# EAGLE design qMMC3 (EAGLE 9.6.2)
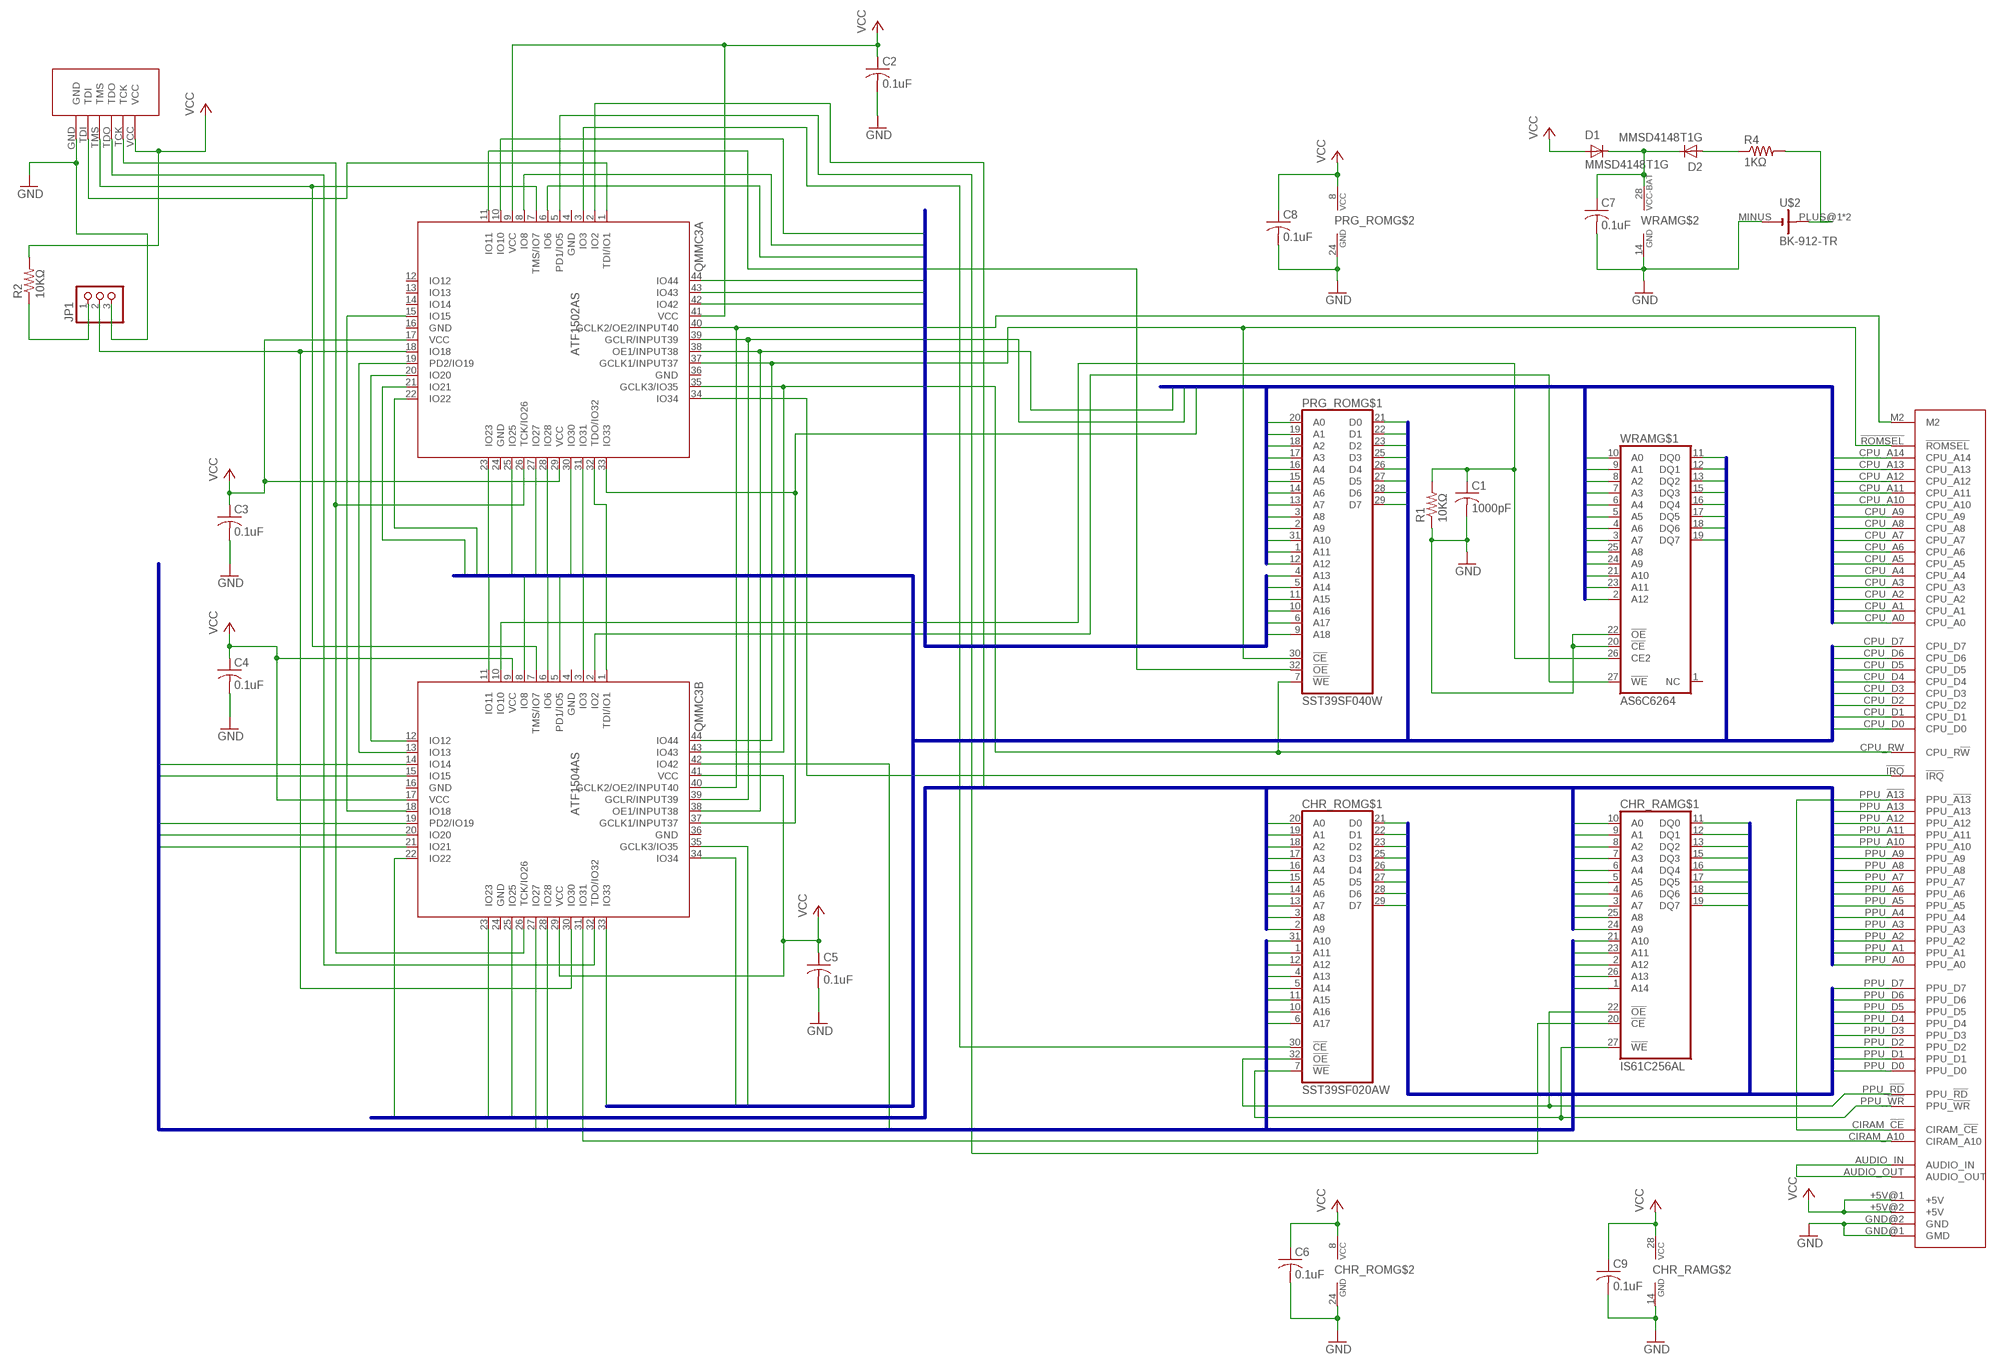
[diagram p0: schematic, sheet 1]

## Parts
C1  1000pF  C-USC1608  [C1608]
C2  0.1uF  C-USC1608  [C1608]
C3  0.1uF  C-USC1608  [C1608]
C4  0.1uF  C-USC1608  [C1608]
C5  0.1uF  C-USC1608  [C1608]
C6  0.1uF  C-USC0603  [C0603]
C7  0.1uF  C-USC1608  [C1608]
C8  0.1uF  C-USC1608  [C1608]
C9  0.1uF  C-USC0603  [C0603]
CHR_RAM  IS61C256AL  [TSOP1-28]
CHR_ROM  SST39SF020AW  [TSOP32S]
D1  MMSD4148T1G  [SOD123FL]
D2  MMSD4148T1G  [SOD123FL]
EDGE1  FC_CARTRIGE_EDGE  [FC_CARTRIDGE_EDGE]
JP1  PINHD-1X3  [1X03]
PRG_ROM  SST39SF040W  [TSOP32S]
QMMC3A  ATF1502AS  [TQFP44]
QMMC3B  ATF1504AS  [TQFP44]
R1  10KΩ  R-US_R0603  [R0603]
R2  10KΩ  R-US_R0603  [R0603]
R4  1KΩ  R-US_R0603  [R0603]
U$1  JTAG_PAD3  [JTAG_PAD3]
U$2  BK-912-TR  [BK-912-TR]
WRAM  AS6C6264  [SOP28]

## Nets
!IRQ: EDGE1.!IRQ QMMC3A.34(IO34)
!ROMSEL: EDGE1.!ROMSEL PRG_ROM.30(!CE) QMMC3A.37(GCLK1/INPUT37) QMMC3B.44(IO44)
_CHR_RAM_CE: CHR_RAM.20(!CE) QMMC3A.5(PD1/IO5)
_CHR_ROM_CE: CHR_ROM.30(!CE) QMMC3A.3(IO3)
AUDIO: EDGE1.AUDIO_IN EDGE1.AUDIO_OUT
BANK_SEL_G: QMMC3A.20(IO20) QMMC3B.12(IO12)
BANK_SEL_H: QMMC3A.19(PD2/IO19) QMMC3B.13(IO13)
CHR_ADDR10: CHR_RAM.21(A10) CHR_ROM.31(A10) QMMC3B.27(IO27)
CHR_ADDR11: CHR_RAM.23(A11) CHR_ROM.1(A11) QMMC3B.42(IO42)
CHR_ADDR12: CHR_RAM.2(A12) CHR_ROM.12(A12) QMMC3B.28(IO28)
CHR_ADDR13: CHR_RAM.26(A13) CHR_ROM.4(A13) QMMC3B.14(IO14)
CHR_ADDR14: CHR_RAM.1(A14) CHR_ROM.5(A14) QMMC3B.15(IO15)
CHR_ADDR15: CHR_ROM.11(A15) QMMC3B.21(IO21)
CHR_ADDR16: CHR_ROM.10(A16) QMMC3B.20(IO20)
CHR_ADDR17: CHR_ROM.6(A17) QMMC3B.19(PD2/IO19)
CHR_SEL: JP1.2 QMMC3A.18(IO18) QMMC3B.30(IO30)
CIRAM_!CE: EDGE1.CIRAM_!CE EDGE1.PPU_!A13
CPU_ADDR0: EDGE1.CPU_A0 PRG_ROM.20(A0) QMMC3A.33(IO33) QMMC3B.37(GCLK1/INPUT37) WRAM.10(A0)
CPU_ADDR1: EDGE1.CPU_A1 PRG_ROM.19(A1) WRAM.9(A1)
CPU_ADDR2: EDGE1.CPU_A2 PRG_ROM.18(A2) WRAM.8(A2)
CPU_ADDR3: EDGE1.CPU_A3 PRG_ROM.17(A3) WRAM.7(A3)
CPU_ADDR4: EDGE1.CPU_A4 PRG_ROM.16(A4) WRAM.6(A4)
CPU_ADDR5: EDGE1.CPU_A5 PRG_ROM.15(A5) WRAM.5(A5)
CPU_ADDR6: EDGE1.CPU_A6 PRG_ROM.14(A6) WRAM.4(A6)
CPU_ADDR7: EDGE1.CPU_A7 PRG_ROM.13(A7) WRAM.3(A7)
CPU_ADDR8: EDGE1.CPU_A8 PRG_ROM.3(A8) WRAM.25(A8)
CPU_ADDR9: EDGE1.CPU_A9 PRG_ROM.2(A9) WRAM.24(A9)
CPU_ADDR10: EDGE1.CPU_A10 PRG_ROM.31(A10) WRAM.21(A10)
CPU_ADDR11: EDGE1.CPU_A11 PRG_ROM.1(A11) WRAM.23(A11)
CPU_ADDR12: EDGE1.CPU_A12 PRG_ROM.12(A12) WRAM.2(A12)
CPU_ADDR13: EDGE1.CPU_A13 QMMC3A.39(GCLR/INPUT39) QMMC3B.39(GCLR/INPUT39)
CPU_ADDR14: EDGE1.CPU_A14 QMMC3A.38(OE1/INPUT38) QMMC3B.38(OE1/INPUT38)
CPU_DATA0: EDGE1.CPU_D0 PRG_ROM.21(D0) QMMC3A.21(IO21) QMMC3B.33(IO33) WRAM.11(DQ0)
CPU_DATA1: EDGE1.CPU_D1 PRG_ROM.22(D1) QMMC3A.22(IO22) QMMC3B.34(IO34) WRAM.12(DQ1)
CPU_DATA2: EDGE1.CPU_D2 PRG_ROM.23(D2) QMMC3A.23(IO23) QMMC3B.35(GCLK3/IO35) WRAM.13(DQ2)
CPU_DATA3: EDGE1.CPU_D3 PRG_ROM.25(D3) QMMC3A.25(IO25) QMMC3B.11(IO11) WRAM.15(DQ3)
CPU_DATA4: EDGE1.CPU_D4 PRG_ROM.26(D4) QMMC3A.27(IO27) QMMC3B.8(IO8) WRAM.16(DQ4)
CPU_DATA5: EDGE1.CPU_D5 PRG_ROM.27(D5) QMMC3A.28(IO28) QMMC3B.6(IO6) WRAM.17(DQ5)
CPU_DATA6: EDGE1.CPU_D6 PRG_ROM.28(D6) QMMC3A.30(IO30) QMMC3B.5(PD1/IO5) WRAM.18(DQ6)
CPU_DATA7: EDGE1.CPU_D7 PRG_ROM.29(D7) QMMC3A.31(IO31) QMMC3B.3(IO3) WRAM.19(DQ7)
CPU_RW: EDGE1.CPU_RW(CPU_R!W) PRG_ROM.7(!WE) QMMC3A.35(GCLK3/IO35) QMMC3B.43(IO43)
GND: C1.2 C2.2 C3.2 C4.2 C5.2 C6.2 C7.2 C8.2 C9.2 CHR_RAM.14(GND) CHR_ROM.24(GND) EDGE1.GND@1(GMD) EDGE1.GND@2(GND) JP1.3 PRG_ROM.24(GND) R1.1 U$1.GND U$2.MINUS(-) WRAM.14(GND) WRAM.20(!CE) WRAM.22(!OE)
HBLANK: QMMC3A.15(IO15) QMMC3B.18(IO18)
M2: EDGE1.M2 QMMC3A.40(GCLK2/OE2/INPUT40) QMMC3B.40(GCLK2/OE2/INPUT40)
N$1: QMMC3A.32(TDO/IO32) QMMC3B.1(TDI/IO1)
N$2: JP1.1 R2.1
N$3: D2.A R4.1
N$4: R4.2 U$2.PLUS@1(+) U$2.PLUS@2(+)
N$44: QMMC3A.1(TDI/IO1) U$1.TDI
N$45: QMMC3A.7(TMS/IO7) QMMC3B.7(TMS/IO7) U$1.TMS
N$46: QMMC3B.32(TDO/IO32) U$1.TDO
N$47: QMMC3A.26(TCK/IO26) QMMC3B.26(TCK/IO26) U$1.TCK
PPU_!RD: CHR_RAM.22(!OE) CHR_ROM.32(!OE) EDGE1.PPU_!RD
PPU_!WR: CHR_RAM.27(!WE) CHR_ROM.7(!WE) EDGE1.PPU_!WR
PPU_ADDR0: CHR_RAM.10(A0) CHR_ROM.20(A0) EDGE1.PPU_A0
PPU_ADDR1: CHR_RAM.9(A1) CHR_ROM.19(A1) EDGE1.PPU_A1
PPU_ADDR2: CHR_RAM.8(A2) CHR_ROM.18(A2) EDGE1.PPU_A2
PPU_ADDR3: CHR_RAM.7(A3) CHR_ROM.17(A3) EDGE1.PPU_A3
PPU_ADDR4: CHR_RAM.6(A4) CHR_ROM.16(A4) EDGE1.PPU_A4
PPU_ADDR5: CHR_RAM.5(A5) CHR_ROM.15(A5) EDGE1.PPU_A5
PPU_ADDR6: CHR_RAM.4(A6) CHR_ROM.14(A6) EDGE1.PPU_A6
PPU_ADDR7: CHR_RAM.3(A7) CHR_ROM.13(A7) EDGE1.PPU_A7
PPU_ADDR8: CHR_RAM.25(A8) CHR_ROM.3(A8) EDGE1.PPU_A8
PPU_ADDR9: CHR_RAM.24(A9) CHR_ROM.2(A9) EDGE1.PPU_A9
PPU_ADDR10: EDGE1.PPU_A10 QMMC3B.25(IO25)
PPU_ADDR11: EDGE1.PPU_A11 QMMC3B.23(IO23)
PPU_ADDR12: EDGE1.PPU_A12 QMMC3B.22(IO22)
PPU_ADDR13: EDGE1.PPU_A13 QMMC3A.2(IO2)
PPU_DATA0: CHR_RAM.11(DQ0) CHR_ROM.21(D0) EDGE1.PPU_D0
PPU_DATA1: CHR_RAM.12(DQ1) CHR_ROM.22(D1) EDGE1.PPU_D1
PPU_DATA2: CHR_RAM.13(DQ2) CHR_ROM.23(D2) EDGE1.PPU_D2
PPU_DATA3: CHR_RAM.15(DQ3) CHR_ROM.25(D3) EDGE1.PPU_D3
PPU_DATA4: CHR_RAM.16(DQ4) CHR_ROM.26(D4) EDGE1.PPU_D4
PPU_DATA5: CHR_RAM.17(DQ5) CHR_ROM.27(D5) EDGE1.PPU_D5
PPU_DATA6: CHR_RAM.18(DQ6) CHR_ROM.28(D6) EDGE1.PPU_D6
PPU_DATA7: CHR_RAM.19(DQ7) CHR_ROM.29(D7) EDGE1.PPU_D7
PRG_ADDR13: PRG_ROM.4(A13) QMMC3A.8(IO8)
PRG_ADDR14: PRG_ROM.5(A14) QMMC3A.6(IO6)
PRG_ADDR15: PRG_ROM.11(A15) QMMC3A.42(IO42)
PRG_ADDR16: PRG_ROM.10(A16) QMMC3A.43(IO43)
PRG_ADDR17: PRG_ROM.6(A17) QMMC3A.10(IO10)
PRG_ADDR18: PRG_ROM.9(A18) QMMC3A.44(IO44)
PRG_CE: PRG_ROM.32(!OE) QMMC3A.11(IO11)
VCC: C2.1 C3.1 C4.1 C5.1 C6.1 C8.1 C9.1 CHR_RAM.28(VCC) CHR_ROM.8(VCC) D1.A EDGE1.+5V@1(+5V) EDGE1.+5V@2(+5V) PRG_ROM.8(VCC) QMMC3A.9(VCC) QMMC3A.17(VCC) QMMC3A.29(VCC) QMMC3A.41(VCC) QMMC3B.9(VCC) QMMC3B.17(VCC) QMMC3B.29(VCC) QMMC3B.41(VCC) R2.2 U$1.VCC
VCC_BAT: C7.1 D1.C D2.C WRAM.28(VCC-BAT)
VRAM_A10: EDGE1.CIRAM_A10 QMMC3B.31(IO31)
WRAM_CE: C1.1 QMMC3B.10(IO10) R1.2 WRAM.26(CE2)
WRAM_WE: QMMC3B.2(IO2) WRAM.27(!WE)
Unconnected: QMMC3A.12(IO12) QMMC3A.13(IO13) QMMC3A.14(IO14) WRAM.1(NC)

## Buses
CPU_ADDR[0..14]
CPU_DATA[0..7]
PPU_ADDR[0..13]
PPU_DATA[0..7]
PRG_ADDR[13..18]
CHR_ADDR[10..17]

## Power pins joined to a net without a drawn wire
GND: QMMC3A.4(GND) QMMC3A.16(GND) QMMC3A.24(GND) QMMC3A.36(GND) QMMC3B.4(GND) QMMC3B.16(GND) QMMC3B.24(GND) QMMC3B.36(GND)

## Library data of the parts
C1-C9 = rcl:C-US: CAPACITOR, American symbol; SPICEPREFIX: C
CHR_RAM = pMMC3:IS61C256AL
CHR_ROM = pMMC3:SST39SF020A: 2 Mbit x8 Multi-Purpose Flash Source: http://ww1.microchip.com/downloads/en/DeviceDoc/20005022C.pdf
D1 D2 = pMMC3:MMSD4148T1G: MMSD4148T1G
EDGE1 = pMMC3:FC_CARTRIGE_EDGE
JP1 = pinhead:PINHD-1X3: PIN HEADER
PRG_ROM = pMMC3:SST39SF040: 4 Mbit x8 Multi-Purpose Flash Source: http://ww1.microchip.com/downloads/en/DeviceDoc/20005022C.pdf
QMMC3A = pMMC3:ATF1502AS
QMMC3B = pMMC3:ATF1504AS
R1 R2 R4 = rcl:R-US_: RESISTOR, American symbol; SPICEPREFIX: R
U$1 = pMMC3:JTAG_PAD3
U$2 = pMMC3:BK-912-TR
WRAM = pMMC3:AS6C6264: AS6C62256 Source; https://www.alliancememory.com/wp-content/uploads/pdf/AS6C62256.pdf

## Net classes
0 default: width 0.254 mm, drill 0.254 mm, clearance 0.127 mm

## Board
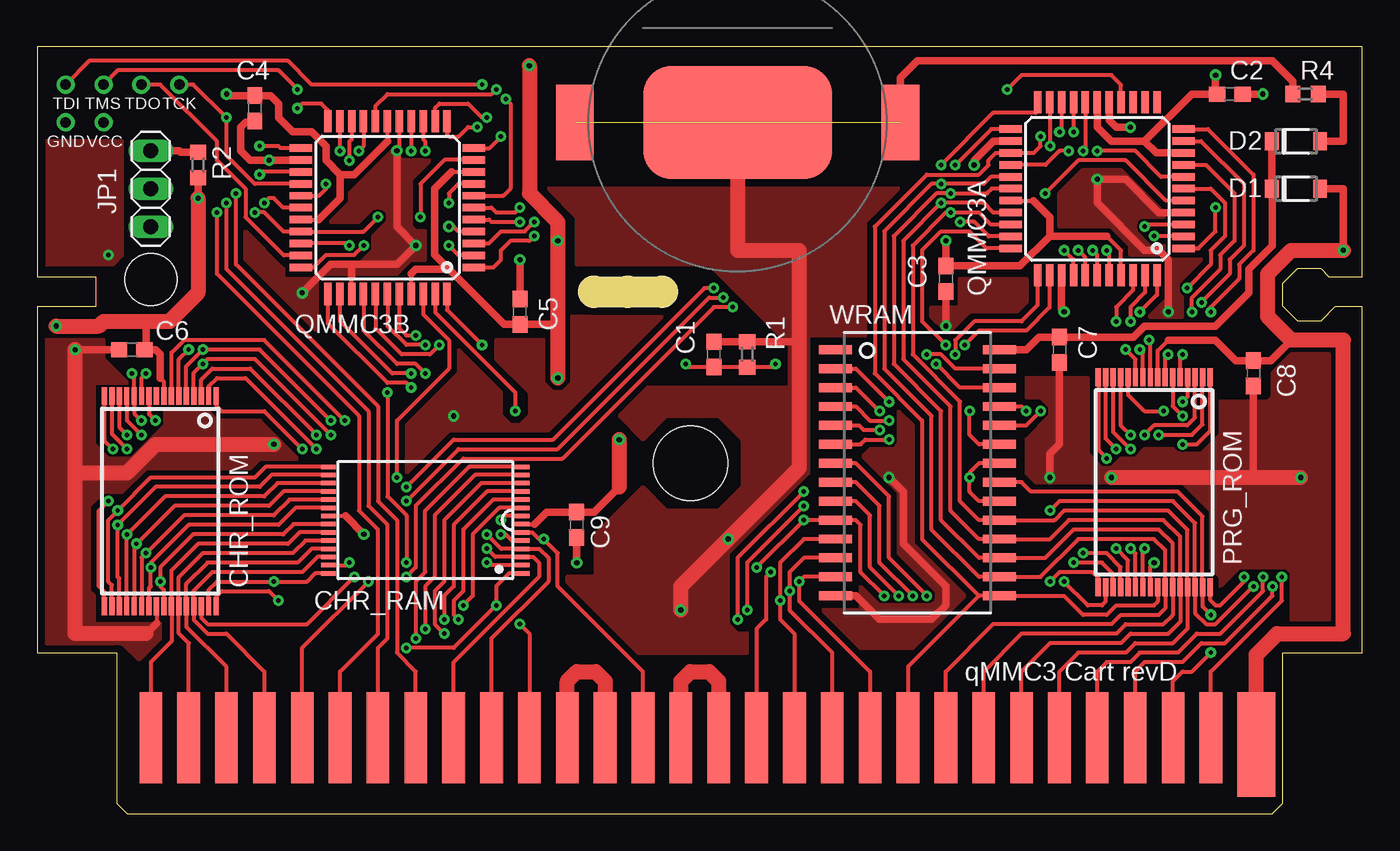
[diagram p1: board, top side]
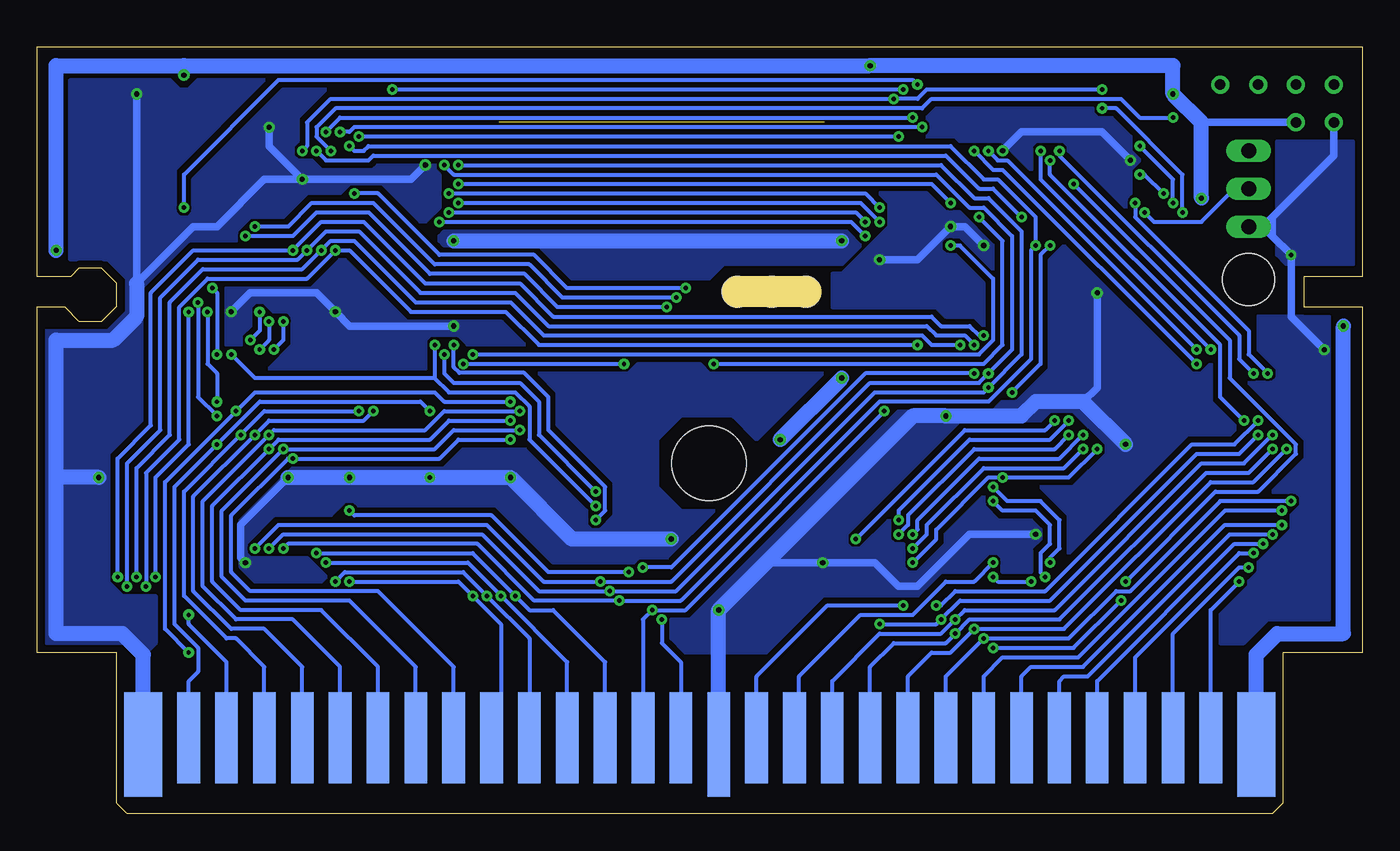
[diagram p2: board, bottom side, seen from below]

Size 88.9 x 51.44 mm. Coordinates in mm from the lower left corner, seen from the top.
Outline: 5.33,0.7 6.03,0 82.87,0 83.57,0.7 83.57,10.79 88.9,10.79 88.9,33.98 87.07,33.98 86.11,33.02 84.58,33.02 83.57,34.04 83.57,35.56 84.58,36.58 86.11,36.58 86.67,36.02 88.9,36.02 88.9,51.44 0,51.44 0,36.02 3.94,36.02 3.94,33.98 0,33.98 0,10.79 5.33,10.79 5.33,0.7
Outline: 37.34,36.02 41.91,36.02 arc-180 41.91,33.98 37.34,33.98 arc-180 37.34,36.02
Copper layers (1*16): Top 0.035mm / dielectric 1.5mm / Bottom 0.035mm
Design rules "default *": minimum track width 6mil, minimum drill 0.3mm, track to track 5mil, track to pad 5mil, pad to pad 5mil, via to via 5mil, smd to smd 5mil, copper to edge 20mil, drill to drill 6mil, minimum pad ring 10mil, minimum via ring 8mil, stop-mask expansion 4mil, vias tented up to drill 0mil, thermal gap 10mil
Holes 2.03 mm at 37.34,35 41.91,35 39.62,35
Holes 5 mm at 43.81,23.5
Holes 3.5 mm at 7.62,35.81
tKeepout: area 11.4,32.1 to 14,34.6; area 3.2,33 to 5.7,35.6; area 74.3,32.1 to 76.8,34.6; area 83.2,35.6 to 85.7,38.1; area 14,31.8 to 16.5,34.3
Milling: 1 lines

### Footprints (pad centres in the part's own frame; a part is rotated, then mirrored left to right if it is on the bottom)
C1608 = smd 1.1 x 1: 1 -0.85,0; 2 0.85,0
C0603 = smd 1.1 x 1: 1 -0.85,0; 2 0.85,0
TSOP1-28 = smd 1 x 0.3: 1 -6.5,-0.275; 2 -6.5,-0.825; 3 -6.5,-1.375; 4 -6.5,-1.925; 5 -6.5,-2.475; 6 -6.5,-3.025; 7 -6.5,-3.575; 8 6.5,-3.575; 9 6.5,-3.025; 10 6.5,-2.475; 11 6.5,-1.925; 12 6.5,-1.375; 13 6.5,-0.825; 14 6.5,-0.275; 15 6.5,0.275; 16 6.5,0.825; 17 6.5,1.375; 18 6.5,1.925; 19 6.5,2.475; 20 6.5,3.025; 21 6.5,3.575; 22 -6.5,3.575; 23 -6.5,3.025; 24 -6.5,2.475; 25 -6.5,1.925; 26 -6.5,1.375; 27 -6.5,0.825; 28 -6.5,0.275
TSOP32S = smd 1.2 x 0.36: 1 -7.05,3.75; 2 -7.05,3.25; 3 -7.05,2.75; 4 -7.05,2.25; 5 -7.05,1.75; 6 -7.05,1.25; 7 -7.05,0.75; 8 -7.05,0.25; 9 -7.05,-0.25; 10 -7.05,-0.75; 11 -7.05,-1.25; 12 -7.05,-1.75; 13 -7.05,-2.25; 14 -7.05,-2.75; 15 -7.05,-3.25; 16 -7.05,-3.75; 17 7.05,-3.75; 18 7.05,-3.25; 19 7.05,-2.75; 20 7.05,-2.25; 21 7.05,-1.75; 22 7.05,-1.25; 23 7.05,-0.75; 24 7.05,-0.25; 25 7.05,0.25; 26 7.05,0.75; 27 7.05,1.25; 28 7.05,1.75; 29 7.05,2.25; 30 7.05,2.75; 31 7.05,3.25; 32 7.05,3.75
SOD123FL = smd 0.91 x 1.22: A 1.625,0; C -1.625,0
FC_CARTRIDGE_EDGE = smd 1.524 x 6.096 bottom: !IRQ 1.27,0; CIRAM_A10 -6.35,0; CPU_A0 6.35,0; CPU_A1 8.89,0; CPU_A2 11.43,0; CPU_A3 13.97,0; CPU_A4 16.51,0; CPU_A5 19.05,0; CPU_A6 21.59,0; CPU_A7 24.13,0; CPU_A8 26.67,0; CPU_A9 29.21,0; CPU_A10 31.75,0; CPU_A11 34.29,0; CPU_RW 3.81,0; PPU_!RD -3.81,0; PPU_A0 -24.13,0; PPU_A1 -21.59,0; PPU_A2 -19.05,0; PPU_A3 -16.51,0; PPU_A4 -13.97,0; PPU_A5 -11.43,0; PPU_A6 -8.89,0; PPU_D0 -26.67,0; PPU_D1 -29.21,0; PPU_D2 -31.75,0; PPU_D3 -34.29,0 | smd 1.524 x 6.096: !ROMSEL 3.81,0; AUDIO_IN 1.27,0; AUDIO_OUT -1.27,0; CIRAM_!CE -6.35,0; CPU_A12 31.75,0; CPU_A13 29.21,0; CPU_A14 26.67,0; CPU_D0 6.35,0; CPU_D1 8.89,0; CPU_D2 11.43,0; CPU_D3 13.97,0; CPU_D4 16.51,0; CPU_D5 19.05,0; CPU_D6 21.59,0; CPU_D7 24.13,0; M2 34.29,0; PPU_!A13 -8.89,0; PPU_!WR -3.81,0; PPU_A7 -11.43,0; PPU_A8 -13.97,0; PPU_A9 -16.51,0; PPU_A10 -19.05,0; PPU_A11 -21.59,0; PPU_A12 -24.13,0; PPU_A13 -26.67,0; PPU_D4 -36.83,0; PPU_D5 -34.29,0; PPU_D6 -31.75,0; PPU_D7 -29.21,0 | smd 2.54 x 6.985 bottom: +5V@1 -37.338,-0.445; GND@1 37.338,-0.445 | smd 2.54 x 6.985: +5V@2 37.338,-0.445 | smd 1.524 x 6.985 bottom: GND@2 -1.27,-0.445
1X03 = drill 1.016 long: 1 -2.54,0; 2 0,0; 3 2.54,0
TQFP44 = smd 1.5 x 0.5: 1 -5.8,4; 2 -5.8,3.2; 3 -5.8,2.4; 4 -5.8,1.6; 5 -5.8,0.8; 6 -5.8,0; 7 -5.8,-0.8; 8 -5.8,-1.6; 9 -5.8,-2.4; 10 -5.8,-3.2; 11 -5.8,-4; 23 5.8,-4; 24 5.8,-3.2; 25 5.8,-2.4; 26 5.8,-1.6; 27 5.8,-0.8; 28 5.8,0; 29 5.8,0.8; 30 5.8,1.6; 31 5.8,2.4; 32 5.8,3.2; 33 5.8,4 | smd 0.5 x 1.5: 12 -4,-5.8; 13 -3.2,-5.8; 14 -2.4,-5.8; 15 -1.6,-5.8; 16 -0.8,-5.8; 17 0,-5.8; 18 0.8,-5.8; 19 1.6,-5.8; 20 2.4,-5.8; 21 3.2,-5.8; 22 4,-5.8; 34 4,5.8; 35 3.2,5.8; 36 2.4,5.8; 37 1.6,5.8; 38 0.8,5.8; 39 0,5.8; 40 -0.8,5.8; 41 -1.6,5.8; 42 -2.4,5.8; 43 -3.2,5.8; 44 -4,5.8
R0603 = smd 1 x 1.1: 1 -0.85,0; 2 0.85,0
JTAG_PAD3 = drill 0.7: GND -3.81,-1.27; TCK 3.81,1.27; TDI -3.81,1.27; TDO 1.27,1.27; TMS -1.27,1.27; VCC -1.27,-1.27
BK-912-TR = smd 12.7 x 7.62: MINUS 0,0 | smd 2.54 x 5.08: PLUS@1 -10.922,0; PLUS@2 10.922,0
SOP28 = smd 0.6 x 2.2: 1 -8.255,-5.5; 2 -6.985,-5.5; 3 -5.715,-5.5; 4 -4.445,-5.5; 5 -3.175,-5.5; 6 -1.905,-5.5; 7 -0.635,-5.5; 8 0.635,-5.5; 9 1.905,-5.5; 10 3.175,-5.5; 11 4.445,-5.5; 12 5.715,-5.5; 13 6.985,-5.5; 14 8.255,-5.5; 15 8.255,5.5; 16 6.985,5.5; 17 5.715,5.5; 18 4.445,5.5; 19 3.175,5.5; 20 1.905,5.5; 21 0.635,5.5; 22 -0.635,5.5; 23 -1.905,5.5; 24 -3.175,5.5; 25 -4.445,5.5; 26 -5.715,5.5; 27 -6.985,5.5; 28 -8.255,5.5

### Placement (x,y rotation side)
C1  45.4,30.8 90 top
C2  80.01,48.26 0 top
C3  60.96,35.88 270 top
C4  14.61,47.31 270 top
C5  32.38,33.66 90 top
C6  6.35,31.11 180 top
C7  68.58,31.11 270 top
C8  81.6,29.53 270 top
C9  36.2,19.37 270 top
CHR_RAM  26.04,19.68 180 top
CHR_ROM  8.26,20.95 270 top
D1  84.45,41.91 0 top
D2  84.45,45.09 0 top
EDGE1  44.45,5.08 0 top
JP1  7.62,41.91 270 top
PRG_ROM  74.93,22.23 270 top
QMMC3A  71.12,41.91 180 top
QMMC3B  23.5,40.64 180 top
R1  47.62,30.8 270 top
R2  10.79,43.5 270 top
R4  85.09,48.26 180 top
U$1  5.71,47.62 0 top
U$2  46.99,46.35 0 top
WRAM  59.05,22.86 270 top

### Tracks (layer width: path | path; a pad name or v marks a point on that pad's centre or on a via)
!IRQ  (via drill 0.3)
  Top 0.254: QMMC3A.34 67.12,34.1 66.04,33.02 62.87,33.02 61.59,31.75 v61.59,30.8 | v51.44,21.59 46.99,17.14 v46.99,13.02
  Bottom 0.254: v61.59,30.8 61.59,29.53 60.96,28.89 56.52,28.89 55.24,27.62 55.24,25.4 v51.44,21.59 | v46.99,13.02 46.99,11.43 45.72,10.16 EDGE1.!IRQ
!ROMSEL  (via drill 0.3)
  Top 0.254: v81.6,15.24 79.06,12.7 78.42,12.7 77.68,13.44 PRG_ROM.30 77.68,19.48 76.2,20.95 68.58,20.95 v67.94,20.32 | EDGE1.!ROMSEL 48.26,12.38 48.9,13.02 48.9,15.88 v49.21,16.19 | QMMC3A.37 69.52,37.16 v68.9,37.78 | QMMC3B.44 27.5,33.78 v29.84,31.43
  Bottom 0.254: v49.21,16.19 54.61,16.19 58.42,20 67.63,20 v67.94,20.32 | v81.6,15.24 81.6,22.86 79.38,25.08 79.38,33.97 77.47,35.88 70.8,35.88 v68.9,37.78 67.94,37.78 63.82,33.66 57.47,33.66 55.24,31.43 v29.84,31.43
_CHR_RAM_CE  (via drill 0.3)
  Top 0.254: CHR_RAM.20 20.79,16.66 v20.95,16.83 | v24.77,21.91 27.94,25.08 34.61,25.08 44.77,35.24 v45.4,35.24 | v67.63,41.59 69.85,43.81 73.03,43.81 75.73,41.11 QMMC3A.5
  Bottom 0.254: v20.95,16.83 20.95,17.14 20.32,17.78 20.32,19.68 21.59,20.95 23.81,20.95 v24.77,21.91 | v45.4,35.24 53.34,35.24 55.56,37.47 61.91,37.47 66.04,41.59 v67.63,41.59
_CHR_ROM_CE  (via drill 0.3)
  Top 0.254: CHR_ROM.30 11.01,13.12 11.43,12.7 18.1,12.7 v21.27,15.88 | v24.77,20.95 28.26,24.45 34.92,24.45 45.09,34.61 v46.04,34.61 | QMMC3A.3 74.44,39.51 v74.3,39.37
  Bottom 0.254: v21.27,15.88 21.59,16.19 21.59,17.46 20.95,18.1 20.95,19.37 21.91,20.32 24.13,20.32 v24.77,20.95 | v46.04,34.61 53.66,34.61 55.88,36.83 62.23,36.83 66.36,40.96 70.48,40.96 72.07,39.37 v74.3,39.37
AUDIO
  Top 1.016: EDGE1.AUDIO_IN 45.72,8.89 45.09,9.53 43.81,9.53 43.18,8.89 EDGE1.AUDIO_OUT
BANK_SEL_G  (via drill 0.3)
  Top 0.254: QMMC3A.20 68.72,45.86 v68.58,45.72 | QMMC3B.12 27.5,45.53 27.62,45.4 28.26,45.4 28.89,46.04 v29.53,46.04
  Bottom 0.254: v68.58,45.72 67.94,45.72 67.63,46.04 v29.53,46.04
BANK_SEL_H  (via drill 0.3)
  Top 0.254: QMMC3A.19 69.52,45.73 v69.53,45.72 | v30.16,46.67 29.84,46.67 28.89,47.62 26.99,47.62 26.7,47.33 QMMC3B.13
  Bottom 0.254: v69.53,45.72 68.58,46.67 v30.16,46.67
CHR_ADDR10  (via drill 0.3)
  Top 0.254: CHR_RAM.21 18.65,16.11 18.1,15.56 v15.88,15.56 12.06,15.56 11.51,15 CHR_ROM.31 | QMMC3B.27 18.9,41.44 19.37,41.91 v19.37,42.23
  Bottom 0.254: v19.37,42.23 8.89,31.75 8.89,29.21 4.45,24.77 4.45,24.13 6.99,21.59 9.84,21.59 v15.88,15.56
CHR_ADDR11  (via drill 0.3)
  Top 0.254: CHR_RAM.23 30.33,16.66 v30.16,16.83 | QMMC3B.42 25.89,33.48 27.62,31.75 27.62,29.84 24.13,26.35 v24.13,22.54 | v17.78,24.45 15.24,26.99 12.38,26.99 12.01,27.36 CHR_ROM.1
  Bottom 0.254: v30.16,16.83 28.57,18.41 28.57,19.05 25.08,22.54 v24.13,22.54 19.68,22.54 v17.78,24.45
CHR_ADDR12  (via drill 0.3)
  Top 0.254: v6.99,26.35 6.5,26.83 CHR_ROM.12 6.5,29.37 v6.35,29.53 | CHR_RAM.2 30.99,20.51 29.21,18.73 29.21,14.61 v28.57,13.97 | QMMC3B.28 16.51,40.64 15.88,41.27 15.56,41.27 v15.24,40.96
  Bottom 0.254: v6.99,26.35 8.57,24.77 11.43,24.77 21.27,14.92 27.3,14.92 28.26,13.97 v28.57,13.97 | v15.24,40.96 15.24,40.01 7.62,32.38 7.62,30.8 v6.35,29.53
CHR_ADDR13  (via drill 0.3)
  Top 0.254: CHR_ROM.4 10.51,29.55 v11.11,30.16 11.43,30.48 14.61,30.48 v19.68,25.4 | QMMC3B.14 25.89,45.23 26.04,45.09 v26.04,44.45 | v31.11,18.73 31.43,18.73 31.86,18.31 CHR_RAM.26
  Bottom 0.254: v31.11,18.73 30.48,19.37 30.48,20 26.04,24.45 20.64,24.45 v19.68,25.4 | v11.11,30.16 24.13,43.18 24.77,43.18 v26.04,44.45
CHR_ADDR14  (via drill 0.3)
  Top 0.254: CHR_RAM.1 31.39,19.96 v31.11,19.68 | v19.68,26.35 14.92,31.11 v11.11,31.11 10.01,30.01 CHR_ROM.5 | QMMC3B.15 25.09,44.46 v25.08,44.45
  Bottom 0.254: v31.11,19.68 31.11,20.32 26.35,25.08 20.95,25.08 v19.68,26.35 | v25.08,44.45 24.45,43.81 23.81,43.81 v11.11,31.11
CHR_ADDR15  (via drill 0.3)
  Top 0.254: CHR_ROM.11 7,29.23 v7.3,29.53 | QMMC3B.21 20.3,44.48 v20.32,44.45
  Bottom 0.254: v7.3,29.53 8.26,30.48 8.26,32.07 20.32,44.13 v20.32,44.45
CHR_ADDR16  (via drill 0.3)
  Top 0.254: QMMC3B.20 21.09,45.23 20.95,45.09 v20.95,43.81 | CHR_ROM.10 7.5,26.79 v7.94,26.35
  Bottom 0.254: v7.94,26.35 9.53,27.94 9.53,31.43 20.95,42.86 v20.95,43.81
CHR_ADDR17  (via drill 0.3)
  Top 0.254: CHR_ROM.6 9.51,30.46 v10.16,31.11 | QMMC3B.19 21.89,44.76 v21.59,44.45
  Bottom 0.254: v21.59,44.45 21.59,42.55 v10.16,31.11
CHR_SEL  (via drill 0.3)
  Top 0.254: QMMC3A.18 70.32,44.6 v70.17,44.45 | v22.86,40.01 21.89,39.04 QMMC3B.30 16.52,39.04 15.24,40.32 v14.61,40.32
  Bottom 0.254: v70.17,44.45 69.53,43.81 66.67,43.81 66.36,44.13 27.94,44.13 25.72,41.91 24.77,41.91 v22.86,40.01 | v14.61,40.32 13.97,39.69 10.79,39.69 8.57,41.91 JP1.2
CIRAM_!CE
  Top 1.016: EDGE1.PPU_!A13 35.56,8.89 36.2,9.53 37.47,9.53 38.1,8.89 EDGE1.CIRAM_!CE
CPU_ADDR0  (via drill 0.3)
  Top 0.254: PRG_ROM.20 72.68,16.54 71.75,17.46 v70.17,17.46 | v56.83,14.61 55.24,16.19 55.24,19.37 54.93,19.68 WRAM.10 v51.44,19.68 v48.26,16.51 | QMMC3A.33 63.69,37.91 62.55,39.05 60.64,39.05 59.37,37.78 59.37,33.02 v60.96,31.43 | QMMC3B.37 21.89,32.4 24.13,30.16 25.4,30.16 v26.04,29.53
  Bottom 0.254: EDGE1.CPU_A0 50.8,10.16 54.29,13.65 55.88,13.65 v56.83,14.61 59.69,17.46 v70.17,17.46 | v51.44,19.68 50.8,20.32 50.8,21.91 54.61,25.72 54.61,27.94 56.23,29.55 60.58,29.55 60.96,29.94 v60.96,31.43 | v26.04,29.53 33.34,29.53 46.35,16.51 v48.26,16.51
CPU_ADDR1  (via drill 0.3)
  Top 0.254: PRG_ROM.19 72.18,16.09 71.44,16.83 v69.53,16.83 | v57.78,14.61 55.88,16.51 55.88,20 54.93,20.95 WRAM.9
  Bottom 0.254: EDGE1.CPU_A1 53.34,10.16 v57.78,14.61 60.01,16.83 v69.53,16.83
CPU_ADDR2  (via drill 0.3)
  Top 0.254: PRG_ROM.18 71.68,14.21 71.44,13.97 70.48,13.97 v68.9,15.56 | v58.74,14.61 56.52,16.83 56.52,20.64 54.93,22.23 WRAM.8
  Bottom 0.254: EDGE1.CPU_A2 55.88,11.75 v58.74,14.61 60.33,16.19 68.26,16.19 v68.9,15.56
CPU_ADDR3  (via drill 0.3)
  Top 0.254: PRG_ROM.17 71.18,15.81 70.8,16.19 68.58,16.19 v67.94,15.56 | v59.69,14.61 57.15,17.14 57.15,21.27 54.93,23.5 WRAM.7
  Bottom 0.254: v67.94,15.56 60.64,15.56 v59.69,14.61 57.78,12.7 57.78,5.71 EDGE1.CPU_A3
CPU_ADDR4  (via drill 0.3)
  Top 0.254: WRAM.6 55.24,24.77 55.56,25.08 v57.15,25.08 | PRG_ROM.16 71.18,24.39 v71.75,23.81
  Bottom 0.254: EDGE1.CPU_A4 60.96,9.84 66.04,14.92 74.61,14.92 75.88,16.19 75.88,20 72.07,23.81 v71.75,23.81 61.91,23.81 60.64,25.08 v57.15,25.08
CPU_ADDR5  (via drill 0.3)
  Top 0.254: v56.52,25.72 55.46,25.72 55.14,26.04 WRAM.5 | PRG_ROM.15 71.68,25.16 v72.39,24.45
  Bottom 0.254: EDGE1.CPU_A5 63.5,9.84 67.94,14.29 74.93,14.29 76.52,15.88 76.52,20.32 v72.39,24.45 62.23,24.45 60.96,25.72 v56.52,25.72
CPU_ADDR6  (via drill 0.3)
  Top 0.254: WRAM.4 54.93,27.3 55.88,26.35 v57.15,26.35 | PRG_ROM.14 72.18,25.61 v73.34,24.45
  Bottom 0.254: EDGE1.CPU_A6 66.04,9.84 69.85,13.65 75.25,13.65 77.15,15.56 77.15,20.64 v73.34,24.45 72.71,25.08 62.55,25.08 61.28,26.35 v57.15,26.35
CPU_ADDR7  (via drill 0.3)
  Top 0.254: WRAM.3 54.93,28.57 v56.52,26.99 | PRG_ROM.13 72.68,26.06 v73.34,25.4
  Bottom 0.254: EDGE1.CPU_A7 68.58,9.84 71.75,13.02 75.56,13.02 77.79,15.24 77.79,20.95 v73.34,25.4 73.03,25.72 62.87,25.72 61.59,26.99 v56.52,26.99
CPU_ADDR8  (via drill 0.3)
  Top 0.254: PRG_ROM.3 77.68,26.56 77.15,26.04 74.93,26.04 v74.3,25.4 | WRAM.25 66.04,27.3 v66.36,26.99
  Bottom 0.254: EDGE1.CPU_A8 71.12,9.84 73.66,12.38 75.88,12.38 78.42,14.92 78.42,21.27 v74.3,25.4 73.34,26.35 66.99,26.35 v66.36,26.99
CPU_ADDR9  (via drill 0.3)
  Top 0.254: PRG_ROM.2 78.18,26.11 77.47,25.4 v75.25,25.4 | WRAM.24 66.36,26.04 v67.31,26.99
  Bottom 0.254: EDGE1.CPU_A9 73.66,9.84 75.56,11.75 76.2,11.75 79.06,14.61 79.06,21.59 v75.25,25.4 73.66,26.99 v67.31,26.99
CPU_ADDR10  (via drill 0.3)
  Top 0.254: v78.74,13.34 78.18,13.89 PRG_ROM.31 78.18,19.93 76.52,21.59 66.67,21.59 66.04,22.23 WRAM.21
  Bottom 0.254: EDGE1.CPU_A10 76.2,10.16 78.74,12.7 v78.74,13.34
CPU_ADDR11  (via drill 0.3)
  Top 0.254: PRG_ROM.1 78.68,25.66 77.79,24.77 v76.83,24.77 | WRAM.23 63.18,24.77 62.55,25.4 v62.55,26.99
  Bottom 0.254: EDGE1.CPU_A11 78.74,8.89 78.11,9.53 78.11,11.11 79.69,12.7 79.69,21.91 v76.83,24.77 73.98,27.62 63.18,27.62 v62.55,26.99
CPU_ADDR12  (via drill 0.3)
  Top 0.254: EDGE1.CPU_A12 76.2,8.89 76.83,9.53 77.47,9.53 v78.74,10.79 | WRAM.2 54.93,29.84 v57.15,27.62 | PRG_ROM.12 73.18,28.1 74.3,26.99 v75.56,26.99
  Bottom 0.254: v78.74,10.79 80.33,12.38 80.33,22.23 v75.56,26.99 74.3,28.26 62.23,28.26 61.59,27.62 v57.15,27.62
CPU_ADDR13  (via drill 0.3)
  Top 0.254: EDGE1.CPU_A13 73.66,9.53 74.3,10.16 76.83,10.16 78.11,11.43 79.69,11.43 82.87,14.61 v82.87,15.24 | QMMC3B.39 23.5,32.7 24.77,31.43 v26.04,31.43 | QMMC3A.39 71.12,37.47 v70.8,37.78
  Bottom 0.254: v82.87,15.24 82.87,23.5 80.64,25.72 80.64,34.61 78.11,37.15 71.44,37.15 v70.8,37.78 69.53,39.05 67.31,39.05 63.18,34.92 56.83,34.92 54.61,32.7 29.21,32.7 28.57,32.07 26.67,32.07 v26.04,31.43
CPU_ADDR14  (via drill 0.3)
  Top 0.254: EDGE1.CPU_A14 71.12,9.53 71.75,10.16 73.34,10.16 73.98,10.79 76.52,10.79 77.79,12.06 79.38,12.06 82.23,14.92 v82.23,15.88 | QMMC3B.38 22.7,32.55 24.45,30.8 26.35,30.8 v26.99,31.43 | QMMC3A.38 70.32,37.31 v69.85,37.78
  Bottom 0.254: v82.23,15.88 82.23,23.18 80.01,25.4 80.01,34.29 77.79,36.51 71.12,36.51 v69.85,37.78 69.22,38.42 67.63,38.42 63.5,34.29 57.15,34.29 54.93,32.07 29.53,32.07 28.89,31.43 v26.99,31.43
CPU_DATA0  (via drill 0.3)
  Top 0.254: EDGE1.CPU_D0 50.8,12.06 49.85,13.02 v49.85,14.29 49.85,16.83 51.44,18.41 WRAM.11 | PRG_ROM.21 73.18,16.99 v72.39,17.78 | QMMC3A.21 67.94,47.69 v67.94,44.77 | QMMC3B.33 18.54,36.64 19.37,37.47 21.27,37.47 v21.91,38.1
  Bottom 0.254: v72.39,17.78 72.07,18.1 59.37,18.1 55.56,14.29 v49.85,14.29 45.72,14.29 32.38,27.62 25.08,27.62 22.23,30.48 22.23,37.78 v21.91,38.1 21.91,40.01 24.45,42.55 25.4,42.55 27.62,44.77 66.67,44.77 66.99,44.45 67.63,44.45 v67.94,44.77
CPU_DATA1  (via drill 0.3)
  Top 0.254: EDGE1.CPU_D1 53.34,10.79 50.48,13.65 v50.48,14.92 50.48,16.19 51.44,17.14 WRAM.12 | PRG_ROM.22 73.68,17.44 v73.34,17.78 | v60.64,43.5 64.14,46.99 66.99,46.99 67.12,47.12 QMMC3A.22 | v25.08,28.57 24.77,28.89 23.5,28.89 19.5,32.89 QMMC3B.34
  Bottom 0.254: v73.34,17.78 72.39,18.73 59.05,18.73 55.24,14.92 v50.48,14.92 46.04,14.92 32.7,28.26 25.4,28.26 v25.08,28.57 22.86,30.8 22.86,39.05 25.08,41.27 26.04,41.27 28.26,43.5 v60.64,43.5
CPU_DATA2  (via drill 0.3)
  Top 0.254: EDGE1.CPU_D2 55.88,9.53 51.12,14.29 v51.12,15.56 51.44,15.88 WRAM.13 | PRG_ROM.23 74.18,17.66 v74.3,17.78 | QMMC3A.23 64.01,45.91 v61.59,43.5 | v25.08,29.53 23.81,29.53 20.3,33.05 QMMC3B.35
  Bottom 0.254: v74.3,17.78 72.71,19.37 58.74,19.37 54.93,15.56 v51.12,15.56 46.35,15.56 33.02,28.89 25.72,28.89 v25.08,29.53 23.5,31.11 23.5,38.73 25.4,40.64 26.35,40.64 28.57,42.86 60.96,42.86 v61.59,43.5
CPU_DATA3  (via drill 0.3)
  Top 0.254: 63.18,14.61 WRAM.15 68.9,14.61 70.17,13.34 71.75,13.34 72.39,13.97 74.93,13.97 75.18,14.22 PRG_ROM.25 | 63.18,14.61 58.42,9.84 EDGE1.CPU_D3 | 63.18,14.61 59.37,18.41 59.37,26.35 56.2,29.53 56.2,39.37 59.69,42.86 63.18,42.86 63.82,43.5 63.82,43.81 64.31,44.31 QMMC3A.25 66.85,44.31 67.31,44.77 v67.31,45.4 | QMMC3B.11 30.35,44.64 v31.11,45.4
  Bottom 0.254: v31.11,45.4 v67.31,45.4
CPU_DATA4  (via drill 0.3)
  Top 0.254: EDGE1.CPU_D4 60.96,9.53 64.14,12.7 72.07,12.7 72.71,13.34 75.25,13.34 75.68,13.77 PRG_ROM.26 75.68,17.66 74.93,18.41 69.85,18.41 67.31,15.88 WRAM.16 63.18,15.88 60.01,19.05 60.01,26.67 56.83,29.84 56.83,39.05 60.01,42.23 v60.64,42.23 63.5,42.23 63.98,42.71 QMMC3A.27 | QMMC3B.8 28.27,42.24 27.62,41.59 v27.62,40.96
  Bottom 0.254: v27.62,40.96 28.89,42.23 v60.64,42.23
CPU_DATA5  (via drill 0.3)
  Top 0.254: EDGE1.CPU_D5 63.5,9.53 66.04,12.06 72.39,12.06 73.03,12.7 75.56,12.7 76.18,13.31 PRG_ROM.27 76.18,18.12 75.25,19.05 69.53,19.05 67.63,17.14 WRAM.17 63.18,17.14 60.64,19.68 60.64,26.99 57.47,30.16 57.47,38.73 60.33,41.59 v61.28,41.59 63.73,41.59 64.05,41.91 QMMC3A.28 | QMMC3B.6 30.48,40.64 30.8,40.32 32.07,40.32 v32.38,40.64
  Bottom 0.254: v61.28,41.59 33.34,41.59 v32.38,40.64
CPU_DATA6  (via drill 0.3)
  Top 0.254: EDGE1.CPU_D6 66.04,9.53 67.94,11.43 72.71,11.43 73.34,12.06 75.88,12.06 76.68,12.86 PRG_ROM.28 76.68,18.57 75.56,19.68 69.22,19.68 67.94,18.41 WRAM.18 63.18,18.41 61.28,20.32 61.28,27.3 58.1,30.48 58.1,38.42 v60.64,40.96 63.5,40.96 64.15,40.31 QMMC3A.30 | QMMC3B.5 30.33,39.84 30.48,39.69 v32.38,39.69
  Bottom 0.254: v32.38,39.69 33.66,40.96 v60.64,40.96
CPU_DATA7  (via drill 0.3)
  Top 0.254: EDGE1.CPU_D7 68.58,9.53 69.85,10.79 73.03,10.79 73.66,11.43 76.2,11.43 77.18,12.41 PRG_ROM.29 77.18,19.02 75.88,20.32 68.9,20.32 68.26,19.68 WRAM.19 63.18,19.68 61.91,20.95 61.91,27.62 58.74,30.8 58.74,38.1 60.96,40.32 v61.28,40.32 63.18,40.32 63.99,39.51 QMMC3A.31 | QMMC3B.3 30.3,38.24 31.11,39.05 32.7,39.05 v33.34,39.69
  Bottom 0.254: v61.28,40.32 33.97,40.32 v33.34,39.69
CPU_RW  (via drill 0.3)
  Top 0.254: PRG_ROM.7 75.68,30.59 v75.88,30.8 | QMMC3A.35 67.92,33.95 66.36,32.38 63.18,32.38 v62.23,31.43 | v51.44,20.64 47.62,16.83 v47.62,13.65 | QMMC3B.43 26.7,33.63 32.07,28.26 v32.07,26.99
  Bottom 0.254: EDGE1.CPU_RW 48.26,13.02 v47.62,13.65 45.4,13.65 v32.07,26.99 | v62.23,31.43 62.23,29.21 | 62.23,29.21 61.28,28.26 56.83,28.26 55.88,27.3 55.88,25.08 v51.44,20.64 | 62.23,29.21 74.3,29.21 v75.88,30.8
GND  (via drill 0.3, 0.35)
  Top 0.254: CHR_ROM.24 8.01,12.77 | CHR_RAM.14 20.68,19.96 | PRG_ROM.24 74.68,16.58 v74.93,16.83 | QMMC3B.4 28.27,39.04 27.94,39.37 v27.62,39.37 | C4.2 14.5,46.35 | QMMC3B.24 17.67,43.81 | QMMC3B.36 21.09,36.02 | QMMC3B.16 24.3,44.62 v24.13,44.45 | WRAM.20 63.18,20.95 62.55,21.59 v62.55,22.54 62.55,22.86 63.18,23.5 WRAM.22 | 51.02,31.65 51.12,31.75
  Top 0.508: 8.01,12.77 7.3,12.06 | 20.68,19.96 v21.91,18.73 | 14.5,46.35 13.97,46.35 13.65,46.04 13.65,44.45 14.29,43.81 v15.56,43.81 17.67,43.81 | v24.13,44.45 24.13,39.37 v25.4,38.1 24.13,36.83 21.27,36.83 | v32.38,37.15 C5.2 | v67.94,22.54 67.94,24.13 68.58,24.77 C7.2 | v57.15,22.54 58.1,21.59 58.1,18.1 60.96,15.24 60.96,13.97 60.01,13.02 56.52,13.02 54.93,14.61 WRAM.14 | C1.2 R1.1 51.02,31.65 | C9.2 v36.2,16.83 | QMMC3A.24 64.16,45.11 62.87,43.81 v62.87,43.5 | QMMC3A.16 71.92,46.51 72.39,46.04 v73.34,46.04 | v75.88,33.66 75.88,37.15 75.25,37.78 74.3,37.78 71.12,40.96 v71.12,42.55 73.03,42.55 75.26,40.31 QMMC3A.4 | QMMC3A.36 68.72,33.83 v68.9,33.66 | C8.2 81.6,22.54 | C2.2 v82.23,48.26 | v2.54,31.11 C6.2 | C3.2 v60.96,32.7 | v17.78,34.92 19.68,36.83 21.27,36.83 | 21.09,36.02 21.09,36.65 21.27,36.83
  Top 1.016: 7.3,12.06 2.54,12.06 2.54,22.86 | 2.54,22.86 v2.54,31.11 | v15.88,24.77 7.94,24.77 6.03,22.86 2.54,22.86 | v72.07,22.54 81.6,22.54 v84.77,22.54 | U$2.MINUS 46.99,37.78 51.12,37.78 51.12,31.75 51.12,23.18 v46.35,18.41 43.18,15.24 v43.18,13.65
  Bottom 0.254: 6.67,39.37 6.99,39.37
  Bottom 0.508: v21.91,18.73 26.35,18.73 29.84,15.24 31.11,15.24 32.7,16.83 v36.2,16.83 40.01,16.83 | v74.93,16.83 75.25,17.14 75.25,19.37 v72.07,22.54 | v15.56,43.81 17.46,45.72 22.86,45.72 v24.13,44.45 | v25.4,38.1 26.67,39.37 v27.62,39.37 29.84,37.15 v32.38,37.15 | v62.87,43.5 63.82,42.55 v71.12,42.55 | v75.88,33.66 74.61,34.92 70.17,34.92 v68.9,33.66 67.94,32.7 v60.96,32.7 | v82.23,48.26 82.23,35.56 78.42,39.37 76.83,39.37 73.66,42.55 v71.12,42.55 | 18.73,27.62 17.78,28.57 v17.78,34.92 | v2.54,31.11 4.76,33.34 v4.76,37.47 6.03,38.73 | JP1.3 6.99,39.37 | 6.03,40.01 6.67,39.37 6.03,38.73 | 6.03,40.01 1.91,44.13 U$1.GND | v71.12,42.55 73.34,44.77 v73.34,46.04 | 6.03,40.01 6.03,38.73
  Bottom 1.016: v15.88,24.77 18.73,27.62 21.91,27.62 22.86,26.67 v27.94,26.67 30.16,26.67 40.01,16.83 v43.18,13.65 EDGE1.GND@2 | EDGE1.GND@1 81.79,10.67 83.19,12.06 87.63,12.06 87.63,22.54 | 87.63,22.54 87.63,31.75 83.82,31.75 82.23,33.34 82.23,35.56 | v72.07,22.54 v67.94,22.54 v62.55,22.54 v57.15,22.54 53.02,18.41 v46.35,18.41 | v84.77,22.54 87.63,22.54
  pour Top: 40.32,10.79 47.62,10.79 47.62,12.06 46.99,12.06 46.35,12.7 46.35,17.46 51.75,22.86 51.75,32.07 55.56,32.07 55.56,39.69 57.78,41.91 34.29,41.91 36.2,40.01 36.2,36.83 45.09,36.83 50.48,31.43 50.48,28.57 40.96,28.57 39.05,26.67 40.64,25.08 42.23,26.67 45.72,26.67 47.31,25.08 47.31,21.91 45.72,20.32 42.23,20.32 40.64,21.91 37.47,18.73 37.47,15.88 35.56,15.88 35.56,15.56
  pour Top: 68.58,39.37 68.58,41.59 70.17,43.18 72.71,43.18 75.56,40.32 75.56,40.01 73.98,40.01 73.66,39.69 73.66,39.05 74.61,38.1 75.56,38.1 75.56,37.47 73.34,37.47 73.34,38.1 72.07,39.37
  pour Top: 74.61,33.34 76.83,33.34 76.83,34.61 76.52,34.92 76.52,35.56 78.11,37.15 75.88,37.15 75.88,34.61
  pour Top: 86.68,30.8 84.14,30.8 82.87,29.53 82.87,27.94 82.55,27.62 79.38,27.62 79.38,25.4 78.11,24.13 76.52,24.13 76.2,24.45 74.3,24.45 73.66,23.81 72.71,23.81 72.07,23.18 71.44,23.18 70.48,24.13 70.48,29.21 66.36,29.21 66.36,27.94 67.31,27.94 67.94,27.3 67.94,26.67 66.36,25.08 66.36,22.86 66.99,22.23 76.83,22.23 78.74,20.32 78.74,16.51 79.38,15.88 79.38,15.24 80.64,16.51 83.82,16.51 84.14,16.19 84.14,13.02 86.68,13.02
  pour Top: 60.01,33.97 61.91,33.97 61.91,35.88 66.36,35.88 66.36,34.29 65.72,33.66 62.55,33.66 61.28,32.38 60.96,32.38 60.01,33.34
  pour Top: 55.4,23.97 57.78,21.59 57.78,17.46 60.33,14.92 60.33,14.29 60.01,13.97 56.52,13.97 55.24,15.24 55.24,13.65 52.7,13.65 55.24,11.11 58.74,11.11 62.23,14.61 58.74,18.1 58.74,26.04 57.78,26.99 57.78,24.77 57.47,24.45 55.88,24.45
  pour Top: 0.64,36.83 5.08,36.83 5.71,37.47 5.71,45.09 0.64,45.09
  pour Bottom: 0.64,36.83 5.08,36.83 5.71,37.47 5.71,38.42 6.35,39.05 6.35,39.69 5.71,40.32 5.71,45.09 0.64,45.09
  pour Bottom: 2.22,33.34 6.99,33.34 6.99,31.11 5.71,29.84 5.71,29.21 6.03,28.89 7.62,28.89 3.81,25.08 3.81,23.81 6.03,21.59 4.45,21.59 4.13,21.27 4.13,20.64 4.76,20 4.76,19.05 6.99,16.83 6.99,16.19 7.62,15.56 7.62,15.24 9.53,13.34 9.53,11.43 7.94,11.43 6.35,13.02 2.22,13.02
  pour Bottom: 43.5,20.32 46.67,17.14 48.58,17.14 48.9,16.83 54.29,16.83 58.1,20.64 67.31,20.64 67.63,20.95 68.26,20.95 69.22,20 73.03,20 74.93,18.1 74.93,17.46 74.61,17.14 70.8,17.14 69.53,15.88 69.85,15.56 74.3,15.56 75.25,16.51 75.25,19.68 71.75,23.18 61.59,23.18 60.33,24.45 56.2,24.45 52.07,20.32 52.07,19.37 51.75,19.05 51.12,19.05 50.16,20 50.16,22.23 53.98,26.04 53.98,28.26 55.24,29.53 49.21,29.53 48.58,30.16 44.45,30.16 43.81,29.53 36.2,29.53 40.64,25.08 42.23,26.67 45.72,26.67 47.31,25.08 47.31,21.91 45.72,20.32
  pour Bottom: 61.91,40.64 62.87,39.69 63.18,39.69 65.72,42.23 67.94,42.23 68.58,41.59 70.8,41.59 72.39,40.01 74.61,40.01 75.56,39.05 75.56,38.42 78.74,38.42 82.87,34.29 82.87,35.88 84.14,37.15 86.68,37.15 86.68,49.21 80.01,49.21 79.38,48.58 78.74,48.58 78.11,49.21 73.66,49.21 79.69,43.18 79.69,40.32 79.38,40.01 78.74,40.01 78.42,40.32 78.42,42.55 72.39,48.58 69.53,48.58 71.44,46.67 71.44,45.09 71.75,44.77 71.75,44.13 71.44,43.81 70.48,43.81 69.85,43.18 66.36,43.18 66.04,43.5 62.23,43.5 62.23,43.18 61.91,42.86
  pour Bottom: 81.92,35.88 81.92,26.35 84.14,24.13 84.14,15.56 83.19,14.61 80.96,14.61 80.96,12.06 80.96,11.43 81.92,10.48 82.87,11.43 88.27,11.43 88.27,32.38 84.14,32.38 82.87,33.66 82.87,35.88
  pour Bottom: 76.2,35.24 70.48,35.24 68.58,37.15 68.26,37.15 64.14,33.02 57.78,33.02 56.2,31.43 60.01,31.43 60.64,32.07 62.55,32.07 62.87,31.75 62.87,29.84 73.34,29.84 71.75,31.43 71.75,33.34 72.07,33.66 73.03,33.66 73.66,34.29 74.3,34.29 74.61,33.97 74.61,32.7 75.25,32.07 75.25,31.43 76.2,31.43
  pour Top: 24.77,26.04 24.77,22.86 27.62,25.72 34.29,25.72 41.91,33.34 35.88,33.34 35.88,28.89 35.24,28.26 34.61,28.26 33.97,28.89 33.97,31.75 30.8,31.75 30.8,30.48 33.02,28.26 33.02,26.67 32.38,26.04 31.75,26.04 31.11,26.67 31.11,28.26 28.26,31.11 28.26,29.53
  pour Top: 19.05,36.2 24.13,36.2 25.08,37.15 25.4,37.15 26.04,37.15 26.04,39.05 25.4,39.05 25.08,39.37 25.08,42.55 26.35,43.81 24.45,43.81 23.81,44.45 20.95,41.59 20.95,40.96 19.68,39.69 21.59,39.69 22.54,40.64 23.18,40.64 23.5,40.32 23.5,39.69 22.54,38.73 22.54,37.78 21.59,36.83 19.68,36.83
  pour Top: 13.97,37.15 13.97,39.05 16.51,36.51 16.51,35.88 18.73,35.88 18.73,32.38
  pour Bottom: 20.95,37.15 20,38.1 11.43,29.53 10.79,29.53 10.16,30.16 10.16,27.62 8.57,26.04 8.57,25.72 8.89,25.4 11.75,25.4 19.68,17.46 19.68,20 21.59,21.91 19.37,21.91 17.14,24.13 17.14,24.77 19.37,26.99 20.95,26.99 21.59,26.35 26.99,26.35 26.35,26.99 24.77,26.99 24.13,27.62 23.18,27.62 20.95,29.84
  pour Bottom: 31.11,26.99 26.35,26.99 34.61,18.73 34.61,18.1 34.29,17.78 33.66,17.78 31.75,19.68 31.75,18.41 31.43,18.1 30.8,18.1 30.8,16.51 30.48,16.19 29.84,16.19 27.94,18.1 27.94,18.73 25.4,21.27 25.4,20.64 24.45,19.68 22.23,19.68 21.59,19.05 21.59,18.41 22.23,17.78 22.23,16.19 24.13,16.19 24.13,17.14 24.45,17.46 25.08,17.46 26.35,16.19 28.26,16.19 29.84,14.61 36.2,14.61 40.01,10.79 45.4,10.79 46.35,11.75 46.35,13.02 45.09,13.02
  pour Bottom: 15.88,40.64 19.68,44.45 19.68,44.77 20,45.09 21.91,45.09 22.23,44.77 22.23,43.18 24.13,45.09 26.99,45.09 27.3,45.4 29.21,45.4 28.89,45.72 28.89,46.35 29.21,46.67 28.57,47.31 18.1,47.31 18.1,46.99 17.78,46.67 16.83,46.67 15.56,45.4 15.56,44.45 14.92,43.81 15.56,43.18 15.56,41.59 15.88,41.27
  pour Bottom: 24.77,36.51 24.77,38.1 26.99,40.32 27.94,40.32 29.21,41.59 32.38,41.59 31.75,40.96 31.75,39.37 34.92,36.2 35.56,36.2 35.56,33.97 28.57,33.97 27.94,33.34 26.04,33.34 25.4,32.7 25.4,35.56 27.3,37.47 27.94,37.47 28.26,37.78 28.26,38.42 27.94,38.73 26.99,38.73
  pour Top: 0.64,11.43 5.71,11.43 6.83,10.32 8.26,11.75 8.26,12.7 3.81,12.7 3.81,14.61 3.49,14.92 3.49,20.64 4.45,21.59 5.71,21.59 7.3,23.18 14.29,23.18 14.92,23.81 17.46,23.81 14.92,26.35 12.06,26.35 11.43,26.99 8.57,26.99 8.57,26.04 6.35,23.81 4.76,23.81 3.81,24.77 3.81,28.89 6.03,28.89 4.45,30.48 4.45,31.75 0.32,31.75 0.64,31.43
HBLANK  (via drill 0.3)
  Top 0.254: v65.09,48.58 66.04,49.53 72.07,49.53 72.72,48.88 QMMC3A.15 | QMMC3B.18 22.7,47.46 23.5,48.26 30.48,48.26 v30.8,48.58
  Bottom 0.254: v65.09,48.58 v30.8,48.58
M2  (via drill 0.3)
  Top 0.254: EDGE1.M2 78.74,9.53 83.5,14.29 v83.5,15.88 | QMMC3A.40 71.92,37.62 v71.75,37.78 | QMMC3B.40 24.3,32.54 24.77,32.07 v25.4,32.07
  Bottom 0.254: v83.5,15.88 83.5,23.81 81.28,26.04 81.28,34.92 78.42,37.78 v71.75,37.78 69.85,39.69 66.99,39.69 62.87,35.56 56.52,35.56 54.29,33.34 28.89,33.34 28.26,32.7 26.35,32.7 25.72,32.07 v25.4,32.07
N$1  (via drill 0.3)
  Top 0.254: QMMC3A.32 63.84,38.71 62.87,39.69 v61.91,39.69 | v33.34,38.73 33.02,38.42 31.75,38.42 31.11,37.78 31.11,37.15 30.61,36.64 QMMC3B.1
  Bottom 0.254: v61.91,39.69 34.29,39.69 v33.34,38.73
N$2
  Top 0.508: R2.1 9.63,44.35 9.53,44.45 JP1.1
N$3
  Top 0.508: R4.1 87.63,48.26 87.63,45.09 D2.A
N$4  (1 unrouted)
  Top 0.508: U$2.PLUS@2 57.91,49.34 59.05,50.48 82.87,50.48 84.24,49.11 R4.2
N$44  (via drill 0.3)
  Top 0.254: QMMC3A.1 77.92,37.91 79.06,39.05 v79.06,40.64 | v29.84,48.9 18.41,48.9 16.83,50.48 3.49,50.48 U$1.TDI
  Bottom 0.254: v79.06,40.64 79.06,42.86 72.71,49.21 30.16,49.21 v29.84,48.9
N$45  (via drill 0.3)
  Top 0.254: QMMC3B.7 31.28,41.44 31.75,41.91 31.75,47.62 v31.43,47.94 | QMMC3A.7 75.4,42.71 73.66,44.45 v71.12,44.45 | v17.46,48.58 16.19,49.85 5.4,49.85 U$1.TMS
  Bottom 0.254: v17.46,48.58 29.21,48.58 29.84,47.94 v31.43,47.94 69.22,47.94 70.8,46.35 70.8,44.77 v71.12,44.45
N$46
  Top 0.254: QMMC3B.32 16.54,37.44 13.97,40.01 13.97,41.91 12.06,43.81 12.06,45.09 8.26,48.9 U$1.TDO
N$47  (via drill 0.3)
  Top 0.254: QMMC3B.26 14.59,42.24 12.7,44.13 v12.7,46.67 10.48,48.9 U$1.TCK | v69.22,44.45 68.58,44.45 67.64,43.51 QMMC3A.26
  Bottom 0.254: v12.7,46.67 14.92,46.67 16.19,47.94 28.89,47.94 29.53,47.31 68.9,47.31 70.17,46.04 70.17,45.4 v69.22,44.45
PPU_!RD  (via drill 0.3)
  Top 0.254: CHR_RAM.22 31.67,16.11 30.8,15.24 v30.8,13.97 27.94,11.11 v24.77,11.11 | CHR_ROM.32 12.01,14.54 12.38,14.92 15.56,14.92 v16.19,14.29
  Bottom 0.254: v30.8,13.97 35.88,13.97 40.64,9.21 EDGE1.PPU_!RD | v24.77,11.11 19.37,11.11 v16.19,14.29
PPU_!WR  (via drill 0.3)
  Top 0.254: EDGE1.PPU_!WR 40.64,9.53 34.92,15.24 34.92,17.46 v33.97,18.41 33.66,18.41 33.21,18.86 CHR_RAM.27 | CHR_ROM.7 9.01,30.91 9.84,31.75 15.24,31.75 v20.64,26.35
  Bottom 0.254: v20.64,26.35 21.27,25.72 26.67,25.72 v33.97,18.41
PPU_ADDR0  (via drill 0.3)
  Top 0.254: CHR_RAM.10 16.13,22.16 15.24,21.27 8.57,21.27 v6.03,18.73 6,18.7 CHR_ROM.20
  Bottom 0.254: EDGE1.PPU_A0 20.32,8.89 20,9.21 18.41,9.21 8.89,18.73 v6.03,18.73
PPU_ADDR1  (via drill 0.3)
  Top 0.254: CHR_RAM.9 15.72,22.71 14.92,21.91 7.94,21.91 v5.4,19.37 5.4,15.88 5.5,15.77 CHR_ROM.19
  Bottom 0.254: EDGE1.PPU_A1 22.86,9.21 22.23,9.84 18.73,9.84 9.21,19.37 v5.4,19.37
PPU_ADDR2  (via drill 0.3)
  Top 0.254: CHR_RAM.8 15.32,23.26 14.61,22.54 7.62,22.54 v5.4,20.32 4.76,19.68 4.76,15.56 5,15.31 CHR_ROM.18
  Bottom 0.254: EDGE1.PPU_A2 25.4,9.21 24.13,10.48 19.05,10.48 9.21,20.32 v5.4,20.32
PPU_ADDR3  (via drill 0.3)
  Top 0.254: CHR_RAM.7 28.98,23.26 26.04,20.32 26.04,16.19 25.4,15.56 v25.4,11.75 | CHR_ROM.17 4.5,14.86 4.13,15.24 4.13,20.32 v4.76,20.95
  Bottom 0.254: EDGE1.PPU_A3 27.94,9.21 v25.4,11.75 19.68,11.75 16.51,14.92 15.56,14.92 9.53,20.95 v4.76,20.95
PPU_ADDR4  (via drill 0.3)
  Top 0.254: CHR_ROM.16 4.5,25.02 v5.08,24.45 | CHR_RAM.6 29.38,22.71 26.67,20 26.67,15.88 26.04,15.24 v26.04,12.38
  Bottom 0.254: EDGE1.PPU_A4 30.48,9.21 28.89,10.79 27.62,10.79 v26.04,12.38 20,12.38 10.16,22.23 7.3,22.23 v5.08,24.45
PPU_ADDR5  (via drill 0.3)
  Top 0.254: CHR_ROM.15 5,25.48 v6.03,24.45 | CHR_RAM.5 29.78,22.16 27.3,19.68 27.3,15.56 26.67,14.92 26.67,12.7 v27.3,12.06
  Bottom 0.254: v6.03,24.45 7.62,22.86 10.48,22.86 20.32,13.02 26.35,13.02 v27.3,12.06 27.94,11.43 31.43,11.43 33.02,9.84 EDGE1.PPU_A5
PPU_ADDR6  (via drill 0.3)
  Top 0.254: CHR_ROM.14 5.5,25.93 v6.03,25.4 | CHR_RAM.4 30.18,21.61 27.94,19.37 27.94,15.24 27.3,14.61 v27.3,13.02
  Bottom 0.254: EDGE1.PPU_A6 35.56,8.89 32.38,12.06 28.26,12.06 v27.3,13.02 26.67,13.65 20.64,13.65 10.79,23.5 7.94,23.5 v6.03,25.4
PPU_ADDR7  (via drill 0.3)
  Top 0.254: CHR_ROM.13 6,26.38 v6.99,25.4 | CHR_RAM.3 30.59,21.06 28.57,19.05 28.57,14.92 27.94,14.29 27.94,13.34 v28.26,13.02 | v32.38,12.7 33.02,12.06 EDGE1.PPU_A7
  Bottom 0.254: v6.99,25.4 8.26,24.13 11.11,24.13 20.95,14.29 26.99,14.29 v28.26,13.02 28.57,12.7 v32.38,12.7
PPU_ADDR8  (via drill 0.3)
  Top 0.254: EDGE1.PPU_A8 30.48,11.75 34.29,15.56 34.29,17.14 33.67,17.76 CHR_RAM.25 31.14,17.76 v30.16,18.73 | CHR_ROM.3 11.01,29.1 11.75,29.84 14.29,29.84 v18.73,25.4
  Bottom 0.254: v30.16,18.73 29.84,19.05 29.84,19.68 25.72,23.81 20.32,23.81 v18.73,25.4
PPU_ADDR9  (via drill 0.3)
  Top 0.254: EDGE1.PPU_A9 27.94,10.16 33.66,15.88 33.66,16.83 33.27,17.21 CHR_RAM.24 30.73,17.21 v30.16,17.78 | CHR_ROM.2 11.51,28.65 12.06,29.21 13.97,29.21 v18.73,24.45
  Bottom 0.254: v30.16,17.78 29.21,18.73 29.21,19.37 25.4,23.18 20,23.18 v18.73,24.45
PPU_ADDR10  (via drill 0.3)
  Top 0.254: EDGE1.PPU_A10 25.4,9.53 24.13,10.79 24.13,19.68 22.86,20.95 22.86,27.3 13.34,36.83 v13.34,41.59 | QMMC3B.25 15.1,43.04 v14.92,42.86
  Bottom 0.254: v14.92,42.86 14.61,42.86 v13.34,41.59
PPU_ADDR11  (via drill 0.3)
  Top 0.254: EDGE1.PPU_A11 22.86,11.11 23.5,11.75 23.5,19.37 22.23,20.64 22.23,26.99 12.7,36.51 v12.7,40.96 | QMMC3B.23 16.32,44.64 16.19,44.77 v14.92,44.77
  Bottom 0.254: v12.7,40.96 12.7,42.55 v14.92,44.77
PPU_ADDR12  (via drill 0.3)
  Top 0.254: EDGE1.PPU_A12 20.32,9.53 22.86,12.06 22.86,19.05 21.59,20.32 21.59,26.67 12.06,36.2 v12.06,40.32 | QMMC3B.22 19.5,47.18 19.05,47.62 17.78,47.62 v17.46,47.31
  Bottom 0.254: v12.06,40.32 12.06,42.86 16.51,47.31 v17.46,47.31
PPU_ADDR13  (via drill 0.3)
  Top 0.254: EDGE1.PPU_A13 17.78,11.11 v22.23,15.56 | v24.77,15.88 25.4,16.51 25.4,20.64 28.57,23.81 35.24,23.81 45.4,33.97 v46.67,33.97 | QMMC3A.2 74.95,38.71 v74.93,38.73
  Bottom 0.254: v24.77,15.88 24.45,15.56 v22.23,15.56 | v46.67,33.97 53.98,33.97 56.2,36.2 62.55,36.2 66.67,40.32 70.17,40.32 71.75,38.73 v74.93,38.73
PPU_DATA0  (via drill 0.3)
  Top 0.254: CHR_ROM.21 6.5,17.93 v6.67,18.1 9.21,20.64 15.56,20.64 16.53,21.61 CHR_RAM.11
  Bottom 0.254: EDGE1.PPU_D0 17.78,8.89 8.57,18.1 v6.67,18.1
PPU_DATA1  (via drill 0.3)
  Top 0.254: CHR_ROM.22 7,17.16 v7.3,17.46 9.84,20 15.88,20 16.93,21.06 CHR_RAM.12
  Bottom 0.254: EDGE1.PPU_D1 15.24,10.48 8.26,17.46 v7.3,17.46
PPU_DATA2  (via drill 0.3)
  Top 0.254: CHR_ROM.23 7.5,15.12 7.62,15.24 v7.62,16.51 7.62,16.83 10.16,19.37 16.19,19.37 17.34,20.51 CHR_RAM.13
  Bottom 0.254: EDGE1.PPU_D2 12.7,12.06 8.26,16.51 v7.62,16.51
PPU_DATA3  (via drill 0.3)
  Top 0.254: CHR_ROM.25 8.51,14.99 8.26,15.24 v8.26,15.56 8.26,16.51 10.48,18.73 16.51,18.73 17.19,19.41 CHR_RAM.15
  Bottom 0.254: EDGE1.PPU_D3 10.16,13.65 v8.26,15.56
PPU_DATA4
  Top 0.254: EDGE1.PPU_D4 7.62,10.16 9.01,11.54 CHR_ROM.26 9.01,16.31 10.79,18.1 16.83,18.1 17.59,18.86 CHR_RAM.16
PPU_DATA5
  Top 0.254: EDGE1.PPU_D5 10.16,11.43 9.51,12.09 CHR_ROM.27 9.51,15.86 11.11,17.46 17.14,17.46 17.99,18.31 CHR_RAM.17
PPU_DATA6
  Top 0.254: EDGE1.PPU_D6 12.7,9.84 10.01,12.54 CHR_ROM.28 10.01,15.4 11.43,16.83 17.46,16.83 18.39,17.76 CHR_RAM.18
PPU_DATA7
  Top 0.254: EDGE1.PPU_D7 15.24,9.53 12.7,12.06 11.43,12.06 10.51,12.99 CHR_ROM.29 10.51,14.95 11.75,16.19 17.78,16.19 18.8,17.21 CHR_RAM.19
PRG_ADDR13  (via drill 0.3)
  Top 0.254: PRG_ROM.4 77.18,27.97 v76.83,27.62 | v77.47,33.66 77.47,34.61 79.38,36.51 79.38,37.47 80.33,38.42 80.33,41.59 78.41,43.51 QMMC3A.8
  Bottom 0.254: v77.47,33.66 77.47,30.16 76.83,29.53 v76.83,27.62
PRG_ADDR14  (via drill 0.3)
  Top 0.254: PRG_ROM.5 76.68,30.64 v76.83,30.8 | v77.15,35.24 78.74,36.83 78.74,37.78 79.69,38.73 79.69,40.96 78.74,41.91 QMMC3A.6
  Bottom 0.254: v77.15,35.24 76.83,34.92 v76.83,30.8
PRG_ADDR15  (via drill 0.3)
  Top 0.254: PRG_ROM.11 73.68,30.46 v73.03,31.11 | QMMC3A.42 73.52,35.1 72.39,33.97 v72.39,33.02
  Bottom 0.254: v73.03,31.11 72.39,31.75 v72.39,33.02
PRG_ADDR16  (via drill 0.3)
  Top 0.254: PRG_ROM.10 74.18,30.91 v73.98,31.11 | QMMC3A.43 74.32,34.95 73.34,33.97 v73.34,33.02
  Bottom 0.254: v73.98,31.11 73.34,31.75 v73.34,33.02
PRG_ADDR17  (via drill 0.3)
  Top 0.254: PRG_ROM.6 76.18,27.32 v76.83,26.67 | v78.11,34.29 80.01,36.2 80.01,37.15 80.96,38.1 80.96,42.23 78.08,45.11 QMMC3A.10
  Bottom 0.254: v76.83,26.67 78.11,27.94 v78.11,34.29
PRG_ADDR18  (via drill 0.3)
  Top 0.254: PRG_ROM.9 74.68,31.68 v74.61,31.75 | QMMC3A.44 75.12,34.8 v73.98,33.66
  Bottom 0.254: v74.61,31.75 73.98,32.38 v73.98,33.66
PRG_CE  (via drill 0.3)
  Top 0.254: v78.74,33.66 78.74,33.97 80.64,35.88 80.64,36.83 81.6,37.78 81.6,42.86 78.55,45.91 QMMC3A.11 | PRG_ROM.32 78.68,14.35 79.06,13.97 79.38,13.97 80.96,15.56 v80.96,15.88
  Bottom 0.254: v80.96,15.88 80.96,22.54 78.74,24.77 v78.74,33.66
VCC  (via drill 0.35)
  Top 0.254: PRG_ROM.8 75.18,31.05 75.88,31.75 | QMMC3A.29 66.84,41.11 | QMMC3A.41 72.72,37.77 71.75,38.73 | 23.5,45.09 QMMC3B.17 | QMMC3B.29 18.89,39.84 | 25.09,36.21 QMMC3B.41 | 27.8,43.04 QMMC3B.9 | CHR_ROM.8 8.51,28.96 8.26,29.21 | C2.1 79.06,48.36 | C6.1 7.3,31.22 | v12.7,48.26 12.8,48.16 | CHR_RAM.28 33.38,19.41 | 34.82,32.8 34.92,32.7
  Top 0.508: 75.88,31.75 79.06,31.75 80.43,30.38 C8.1 82.77,30.38 84.14,31.75 | 67.94,38.73 67.94,40.01 66.84,41.11 | 71.75,38.73 67.94,38.73 | 20.32,42.86 19.37,43.81 19.37,44.77 18.41,45.72 17.14,45.72 16.19,46.67 16.19,47.62 15.66,48.16 C4.1 12.8,48.16 | 23.5,45.09 21.27,42.86 20.32,42.86 | 18.89,39.84 20.32,41.27 20.32,42.86 | 27.62,36.51 25.4,36.51 25.09,36.21 | 27.8,43.04 26.67,41.91 26.67,37.47 27.62,36.51 | QMMC3A.9 75.07,44.31 74.3,45.09 | 74.3,45.09 72.07,45.09 71.12,46.04 QMMC3A.17 | C6.1 7.94,31.11 8.26,30.8 8.26,29.21 | 27.62,36.51 31.33,32.8 C5.1 34.82,32.8 | 67.94,38.73 65.94,36.73 C3.1 v60.96,38.42 | D1.A 87.63,41.91 v87.63,37.78 | 79.06,48.36 v79.06,49.53 | C2.1 77.47,48.26 74.3,45.09 | 7.3,31.22 7.3,33.02 | 39.05,21.91 37.36,20.22 C9.1 34.19,20.22 33.38,19.41 | R2.2 v10.79,41.27
  Top 1.016: v1.27,32.7 4.13,32.7 4.45,33.02 7.3,33.02 8.89,33.02 10.79,34.92 v10.79,41.27 | EDGE1.+5V@2 81.79,10.67 83.19,12.06 87.63,12.06 87.63,31.75 84.14,31.75 82.55,33.34 82.55,36.2 84.14,37.78 v87.63,37.78 | v33.02,50.16 33.02,41.59 34.92,39.69 v34.92,38.42 34.92,32.7 v34.92,29.21 | 39.05,21.91 v39.05,25.08
  Bottom 0.508: v79.06,49.53 79.06,50.16 | U$1.VCC 10.79,46.35
  Bottom 1.016: EDGE1.+5V@1 7.11,10.67 5.71,12.06 1.27,12.06 v1.27,32.7 | v87.63,37.78 87.63,50.16 79.06,50.16 v33.02,50.16 12.7,50.16 v12.7,48.26 10.79,46.35 v10.79,41.27 | v60.96,38.42 v34.92,38.42 | v39.05,25.08 v34.92,29.21
  pour Bottom: 33.66,38.1 34.92,36.83 42.86,36.83 43.81,35.88 53.02,35.88 55.24,38.1 61.59,38.1 61.91,38.42 61.91,38.73 61.59,39.05 34.61,39.05
VCC_BAT
  Top 0.254: 82.87,41.87 D1.C
  Top 0.508: WRAM.28 66.36,31.11 67.21,31.96 C7.1 73.56,31.96 74.3,32.7 79.06,32.7 81.28,34.92 81.28,36.51 82.87,38.1 82.87,41.87 | D1.C D2.C
VRAM_A10  (via drill 0.3)
  Top 0.254: v23.5,28.26 23.5,21.27 24.77,20 v24.77,16.83 | v20.95,38.1 20.82,38.24 QMMC3B.31
  Bottom 0.254: EDGE1.CIRAM_A10 37.78,5.4 37.78,9.21 33.66,13.34 30.16,13.34 27.94,15.56 26.04,15.56 v24.77,16.83 | v20.95,38.1 21.59,37.47 21.59,30.16 v23.5,28.26
WRAM_CE  (via drill 0.3)
  Top 0.254: WRAM.26 61.91,28.57 v60.33,30.16 | v49.53,30.16 49.31,29.95 R1.2 C1.1 43.71,29.95 v43.5,30.16 | QMMC3B.10 27.33,43.84 25.72,42.23 v25.72,40.01
  Bottom 0.254: v60.33,30.16 v49.53,30.16 | v43.5,30.16 25.4,30.16 24.13,31.43 24.13,38.42 v25.72,40.01
WRAM_WE  (via drill 0.3)
  Top 0.254: WRAM.27 61.59,29.84 60.64,30.8 v59.69,30.8 | QMMC3B.2 28.28,37.44 v27.62,38.1
  Bottom 0.254: v59.69,30.8 25.72,30.8 24.77,31.75 24.77,35.88 26.99,38.1 v27.62,38.1

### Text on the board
tPlace: qMMC3 Cart revD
